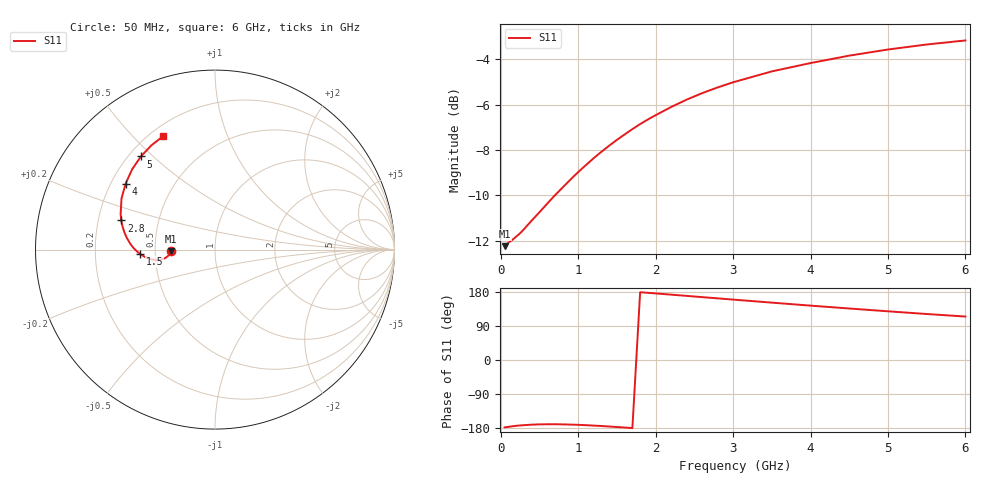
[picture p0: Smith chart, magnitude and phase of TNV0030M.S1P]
! SIEMENS Discrete & RF Semiconductors
! BAS70-07W
! Si Schottky Diode in SOT343
! IF = 30 mA
! S-Parameters:  February  1997
# GHz  S  MA  R  50
!  f  S11
! GHz  MAG  ANG
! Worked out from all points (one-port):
!   34 points, 50 MHz to 6 GHz, reference 50 ohm
!   lowest |S11| = -12.2 dB at 50 MHz (marker M1), VSWR 1.65, Z = 30.4 - j0.578 ohm
!   |S11| at or under -10 dB: start of sweep to 698.7 MHz
!   S11 on the Smith chart (normalised r, x): 50 MHz: 0.61, -0.01; 1.5 GHz: 0.41, -0.02; 2.8 GHz: 0.30, +0.14; 4 GHz: 0.26, +0.31; 5 GHz: 0.25, +0.46; 6 GHz: 0.25, +0.61
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0.05  0.2444 -177.9
0.1  0.249 -176.4
0.15  0.2523 -174.9
0.25  0.261 -172.7
0.4  0.2783 -170.6
0.5  0.2903 -169.9
0.6  0.3033 -169.6
0.7  0.3164 -169.5
0.8  0.3293 -169.9
0.9  0.3427 -170.4
1  0.356 -171.1
1.1  0.3688 -172.0
1.3  0.3946 -174.2
1.5  0.4192 -176.8
1.6  0.431 -178.2
1.8  0.4542 178.8
2  0.4752 175.7
2.2  0.4953 172.5
2.4  0.5141 169.2
2.6  0.5314 165.9
2.8  0.5471 162.7
3  0.5616 159.4
3.5  0.5935 151.4
4  0.6191 143.5
4.5  0.6429 135.9
5  0.6632 128.5
5.5  0.6803 121.4
6  0.6944 114.7
